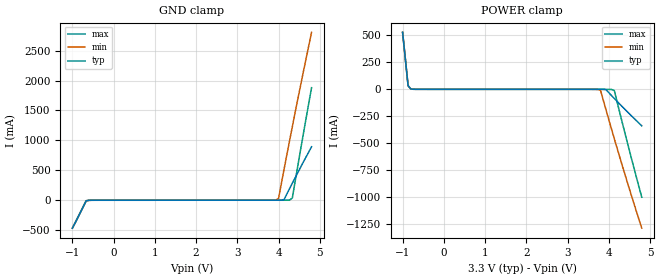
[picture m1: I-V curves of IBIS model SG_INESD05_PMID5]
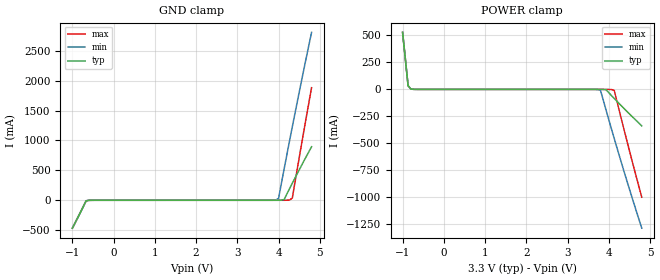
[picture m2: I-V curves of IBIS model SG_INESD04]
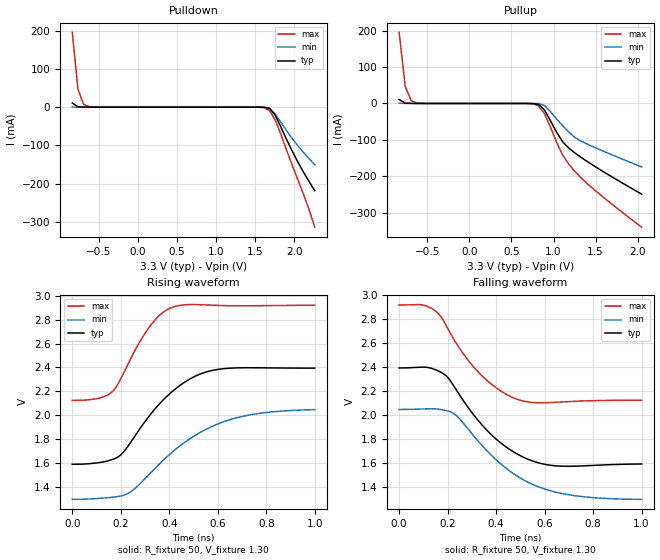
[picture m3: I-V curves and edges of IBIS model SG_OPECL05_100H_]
|   This file is an IBIS representation of the   |
|   Integrated Device Technology , Inc.   |
|   ICS853S310I   |
|   LOW SKEW 1-TO-8 DIFFERNTIAL-TO-3.3V LVPECL/ECL FANOUT BUFFER   |
[IBIS Ver]   4.1
[File name]   853s310i_3v3.ibs
[File Rev]   1.0
[Date]   29 Mar 2011
[Source]   Originated at Integrated Device Technology, Inc.
[Disclaimer]
IDT hereby grants the user of this IBIS model a non-exclusive,
nontransferable license to use this IBIS model under the following terms.
Before using this IBIS model, the user should read this license.
If the user does not accept these terms,  the IBIS model should be
returned to IDT within 30 days.
   The user is granted this license only to use the IBIS model and
is not granted rights to sell, load, rent, lease or license the IBIS
model in whole or in part, or in modified form to anyone other than
user. User may modify the IBIS model to suit its specific
applications but rights to derivative works and such modifications
shall belong to IDT.
   This IBIS model is provided on an "AS IS" basis and IDT makes
absolutely no warranty with respect to the information contained
herein. IDT DISCLAIMS AND CUSTOMER WAIVES ALL WARRANTIES, EXPRESS
OR IMPLIED, INCLUDING WARRANTIES OF MERCHANTABILITY OR FITNESS FOR
A PARTICULAR PURPOSE. The entire risk as to quality and performance
is with the Customer. ACCORDINGLY, IN NO EVENT SHALL THE COMPANY BE
LIABLE FOR ANY DAMAGES, WHETHER IN CONTRACT OR TORT,INCLUDING ANY
LOST PROFITS OR OTHER INCIDENTAL, CONSEQUENTIAL, EXEMPLARY, OR
PUNITIVE DAMAGES ARISING OUT OF THE USE OR APPLICATION OF THE IBIS
model provided in this package. Further, IDT reserves the right to
make changes without notice to any product herein to improve
reliability, function, or design. IDT does not convey any license
under patent rights or any other intellectual property rights,
including those of third parties.
   IDT is not obligated to provide maintenance or support
for the licensed IBIS model.
[Copyright]   Copyright 2011 by Integrated Device Technology , Inc.
[Component]   ICS53S310VI
[Manufacturer] Integrated Device Technology, Inc.
[Package]
|PLCC 28 Pin
|   typ   min   max
R_pkg   53.15m   49.2m   57.1m
L_pkg   3.123nH   2.878nH   3.368nH
C_pkg   0.65pF   0.632pF   0.667pF
[Pin] signal_name   model_name   R_pin   L_pin   C_pin
1   VCC   POWER   49.2m   2.878n   0.632p
2   nPCLK0   SG_INESD05_PMID5   51.2m   3.038n   0.643p
3   VBB   SG_INESD04   53.8m   3.201n   0.655p
4   PCLK1   SG_INESD05_PD75K   57.1m   3.368n   0.667p
5   nPCLK1   SG_INESD05_PMID5   57.1m   3.368n   0.667p
6   NC   NC   53.8m   3.201n   0.655p
7   nQ7   SG_OPECL05_100H_   51.2m   3.038n   0.643p
8   VCCO   POWER   49.2m   2.878n   0.632p
9   Q7   SG_OPECL05_100H_   51.2m   3.038n   0.643p
10   nQ6   SG_OPECL05_100H_   53.8m   3.201n   0.655p
11   Q6   SG_OPECL05_100H_   57.1m   3.368n   0.667p
12   nQ5   SG_OPECL05_100H_   57.1m   3.368n   0.667p
13   Q5   SG_OPECL05_100H_   53.8m   3.201n   0.655p
14   nQ4   SG_OPECL05_100H_   51.2m   3.038n   0.643p
15   VCCO   POWER   49.2m   2.878n   0.632p
16   Q4   SG_OPECL05_100H_   51.2m   3.038n   0.643p
17   nQ3   SG_OPECL05_100H_   53.8m   3.201n   0.655p
18   Q3   SG_OPECL05_100H_   57.1m   3.368n   0.667p
19   nQ2   SG_OPECL05_100H_   57.1m   3.368n   0.667p
20   Q2   SG_OPECL05_100H_   53.8m   3.201n   0.655p
21   nQ1   SG_OPECL05_100H_   51.2m   3.038n   0.643p
22   VCCO   POWER   49.2m   2.878n   0.632p
23   Q1   SG_OPECL05_100H_   51.2m   3.038n   0.643p
24   nQ0   SG_OPECL05_100H_   53.8m   3.201n   0.655p
25   Q0   SG_OPECL05_100H_   57.1m   3.368n   0.667p
26   VEE   GND   57.1m   3.368n   0.667p
27   CLK_SEL   SG_INESD05_PD75K   53.8m   3.201n   0.655p
28   PCLK0   SG_INESD05_PD75K   51.2m   3.038n   0.643p
[Diff Pin]  inv_pin  vdiff tdelay_typ tdelay_min  tdelay_max
|Input
28   2   0.15   0   0   0
4   5   0.15   0   0   0
|Output
9   7   NA   0   0   0
11   10   NA   0   0   0
13   12   NA   0   0   0
16   14   NA   0   0   0
18   17   NA   0   0   0
20   19   NA   0   0   0
23   21   NA   0   0   0
25   24   NA   0   0   0
| Models and submodels in the file (4): SG_INESD05_PMID5 (Input), SG_INESD04 (Input), SG_INESD05_PD75K (Input), SG_OPECL05_100H_ (Output_ECL)
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[Model]   SG_INESD05_PMID5
Model_type   Input
Polarity   Non-Inverting
Vinl = 0.8V
Vinh = 2.0V
|   typ   min   max
C_comp   2pF   1.5pF   2.5pF
|   typ   min   max
[Voltage range]   3.3V   3.135V   3.465V
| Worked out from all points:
|   GND clamp passes 1 mA (typ) near -0.57 V on its own axis
|   POWER clamp passes 1 mA (typ) near -0.75 V on its own axis
[GND_clamp]
|Voltage   I (typ)   I (min)   I (max)
-999mV    -466.2mA   -466.2mA   -466.2mA
-665.7mV  -9.075mA   -9.072mA   -9.078mA
-599.1mV  -1.392mA   -1.388mA   -1.395mA
3.867V    93.26uA    433uA      84.15uA
3.933V    121.1uA    2.991mA    87.1uA
4V        242.2uA    32.96mA    91.88uA
4.133V    10.39mA    518.4mA    165.1uA
4.267V    194mA      994.2mA    3.355mA
4.333V    284.5mA    1.229A     37.1mA
4.533V    550.4mA    1.918A     843mA
4.8V      892.8mA    2.805A     1.88A
[Power_clamp]
|Voltage   I (typ)   I (min)   I (max)
-999mV    527.8mA    527.8mA    527.8mA
-865.7mV  33.62mA    33.62mA    33.63mA
-799mV    3.051mA    3.048mA    3.054mA
3.6V      -77.29uA   -152.7uA   -73.6uA
3.8V      -251uA     -8.905mA   -82.96uA
3.933V    -3.316mA   -190.6mA   -165.6uA
4.133V    -84.48mA   -456.4mA   -9.953mA
4.467V    -214.4mA   -882mA     -517.4mA
4.8V      -338mA     -1.287A    -999.9mA
[Model]   SG_INESD04
Model_type   Input
Polarity   Non-Inverting
Vinl = 0.8V
Vinh = 2.0V
|   typ   min   max
C_comp   2pF   1.5pF   2.5pF
|   typ   min   max
[Voltage range]   3.3V   3.135V   3.465V
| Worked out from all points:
|   GND clamp passes 1 mA (typ) near -0.58 V on its own axis
|   POWER clamp passes 1 mA (typ) near -0.74 V on its own axis
[GND_clamp]
|Voltage   I (typ)   I (min)   I (max)
-999mV    -466.1mA   -466.1mA   -466.1mA
-665.7mV  -8.992mA   -8.992mA   -8.992mA
-599.1mV  -1.311mA   -1.311mA   -1.311mA
3.867V    60.84uA    520.1uA    51.14uA
3.933V    102.7uA    3.239mA    52.58uA
4V        278.2uA    33.38mA    57.05uA
4.133V    10.74mA    519.3mA    166.7uA
4.267V    194.7mA    995.5mA    3.61mA
4.333V    285.4mA    1.23A      37.53mA
4.533V    551.8mA    1.92A      844.1mA
4.8V      894.9mA    2.808A     1.882A
[Power_clamp]
|Voltage   I (typ)   I (min)   I (max)
-999mV    528.7mA    528.7mA    528.7mA
-865.7mV  34.05mA    34.05mA    34.05mA
-799mV    3.3mA      3.298mA    3.302mA
3.6V      -4.407uA   -78.79uA   -1.786uA
3.8V      -172.9uA   -8.826mA   -5.914uA
3.933V    -3.234mA   -190.5mA   -85.07uA
4.133V    -84.39mA   -456.3mA   -9.868mA
4.467V    -214.3mA   -881.9mA   -517.3mA
4.8V      -337.9mA   -1.287A    -999.8mA
[Model]   SG_OPECL05_100H_
Model_type   Output_ECL
Polarity   Non-Inverting
|   typ   min   max
C_comp   2pF   1.5pF   2.5pF
Vmeas = 1.99V
Rref = 50
Cref = 0
Vref = 1.3V
|   typ   min   max
[Voltage range]   3.3V   3.0V   3.8V
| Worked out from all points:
|   rising waveform, R_fixture 50, V_fixture 1.30: 20-80 % time 200ps typ, 277ps min, 132ps max; typ from 1.59 V to 2.4 V
|   falling waveform, R_fixture 50, V_fixture 1.30: 20-80 % time 200ps typ, 245ps min, 175ps max; typ from 2.39 V to 1.59 V
[Pulldown]
|Voltage   I (typ)   I (min)   I (max)
|Note, modeling breaks down at 250mA and above.  This is well beyond the functional   |
|operating range of the device.  Should this scenario occur, catastrophic failure and   |
|possible damage to the device and/or board is of higher concern than the I-V curve   |
|behavior.  The IBIS checker will flag currents in excess of 10A with warnings.  Lines   |
|with currents in excess of 0.35 A have been commented out.  The points still remain|
|available to the user if the user desires to use them.   |
|-3.04000e+00   1.92160e+08   2.51398e+08   1.39180e+08
|-2.78000e+00   1.62857e+08   2.13925e+08   1.17236e+08
|-2.52000e+00   1.33553e+08   1.76452e+08   9.52926e+07
|-2.26000e+00   1.04250e+08   1.38979e+08   7.33492e+07
|-2.00000e+00   7.49467e+07   1.01507e+08   5.14057e+07
|-1.99000e+00   7.38197e+07   1.00065e+08   5.05617e+07
|-1.91789e+00   6.56924e+07   8.96722e+07   4.44757e+07
|-1.84578e+00   5.75651e+07   7.92791e+07   3.83896e+07
|-1.77367e+00   4.94378e+07   6.88860e+07   3.23036e+07
|-1.70156e+00   4.13105e+07   5.84929e+07   2.62176e+07
|-1.62944e+00   3.31832e+07   4.80998e+07   2.01315e+07
|-1.55733e+00   2.50559e+07   3.77067e+07   1.40455e+07
|-1.48522e+00   1.69286e+07   2.73136e+07   7.95945e+06
|-1.41311e+00   8.80127e+06   1.69204e+07   2.03437e+06
|-1.34100e+00   1.34441e+06   6.52733e+06   2.48679e+05
|-1.26889e+00   8.12123e+04   2.80322e+05   3.04058e+04
|-1.19678e+00   4.91291e+03   7.75053e+03   3.72350e+03
|-1.12467e+00   3.01766e+02   2.18996e+02   4.60136e+02
|-1.05256e+00   2.05721e+01   7.44005e+00   5.93641e+01
|-9.80444e-01   1.45327e+00   2.48419e-01   8.49910e+00
|-9.08333e-01   1.25370e-01   8.96926e-03   1.15041e+00
-836.2mV  10.8mA     577.1uA    195.6mA
-764.1mV  1.014mA    102.6uA    46.98mA
-692mV    176.3uA    15.79uA    7.416mA
-619.9mV  34.19uA    1.702uA    1.157mA
1.543V    -16.52uA   -3.526uA   -181.8uA
1.616V    -258uA     -119.7uA   -1.382mA
1.688V    -3.483mA   -3.021mA   -8.864mA
1.76V     -21.46mA   -18.23mA   -33.6mA
1.832V    -52.26mA   -39.77mA   -71.71mA
2.048V    -143.4mA   -100.9mA   -189.5mA
2.192V    -194.7mA   -134.8mA   -268.5mA
2.265V    -218.1mA   -150.1mA   -313.8mA
| 2.33667e+00   -2.40431e-01   -1.64458e-01   -3.51948e-01
| 2.40878e+00   -2.60096e-01   -1.78057e-01   -3.86031e-01
| 2.48089e+00   -2.75926e-01   -1.90995e-01   -4.18389e-01
| 2.55300e+00   -2.90872e-01   -2.03400e-01   -4.50878e-01
| 2.62511e+00   -3.06643e-01   -2.14939e-01   -4.86417e-01
| 2.69722e+00   -3.23573e-01   -2.24622e-01   -5.12879e-01
| 2.76933e+00   -3.40823e-01   -2.33508e-01   -5.36910e-01
| 2.84144e+00   -3.57624e-01   -2.42318e-01   -5.60796e-01
| 2.91356e+00   -3.74840e-01   -2.51157e-01   -5.84860e-01
| 2.98567e+00   -3.92569e-01   -2.59837e-01   -6.08707e-01
| 3.05778e+00   -4.11772e-01   -2.68668e-01   -6.31533e-01
| 3.12989e+00   -4.26759e-01   -2.77928e-01   -6.53567e-01
| 3.20200e+00   -4.40899e-01   -2.86756e-01   -6.74897e-01
| 3.27411e+00   -4.55086e-01   -2.94483e-01   -6.95545e-01
| 3.34622e+00   -4.69164e-01   -3.01542e-01   -7.15540e-01
| 3.41833e+00   -4.82474e-01   -3.08477e-01   -7.34920e-01
| 3.49044e+00   -4.95288e-01   -3.15388e-01   -7.53730e-01
| 3.56256e+00   -5.07746e-01   -3.22427e-01   -7.72015e-01
| 3.63467e+00   -5.19904e-01   -3.29804e-01   -7.89818e-01
| 3.70678e+00   -5.31807e-01   -3.37709e-01   -8.07182e-01
| 3.77889e+00   -5.43539e-01   -3.52649e-01   -8.24146e-01
| 3.85100e+00   -5.55315e-01   -6.12529e-01   -8.40745e-01
| 3.92311e+00   -5.68261e-01   -8.64765e+00   -8.57014e-01
| 3.99522e+00   -5.99695e-01   -2.26919e+02   -8.72983e-01
| 4.06733e+00   -9.36993e-01   -8.00131e+03   -8.88690e-01
| 4.13944e+00   -6.03122e+00   -2.89295e+05   -9.04232e-01
| 4.21156e+00   -6.69016e+01   -1.76555e+06   -9.20172e-01
| 4.28367e+00   -1.03050e+03   -3.81856e+06   -9.40696e-01
| 4.35578e+00   -1.69373e+04   -1.33751e+07   -9.99273e-01
| 4.42789e+00   -2.80216e+05   -2.52525e+07   -1.36920e+00
| 4.50000e+00   -1.41833e+06   -3.71298e+07   -4.27555e+00
| 4.51000e+00   -1.58193e+06   -3.87769e+07   -5.29764e+00
| 4.92800e+00   -4.13220e+07   -1.07625e+08   -5.40432e+05
| 5.34600e+00   -9.51608e+07   -1.76474e+08   -1.86671e+07
| 5.76400e+00   -1.49000e+08   -2.45322e+08   -5.89836e+07
| 6.18200e+00   -2.02838e+08   -3.14171e+08   -9.93001e+07
| 6.60000e+00   -2.56677e+08   -3.83019e+08   -1.39617e+08
[Pullup]
|Voltage   I (typ)   I (min)   I (max)
|Note, modeling breaks down at 250mA and above.  This is well beyond the functional   |
|operating range of the device.  Should this scenario occur, catastrophic failure and   |
|possible damage to the device and/or board is of higher concern than the I-V curve   |
|behavior.  The IBIS checker will flag currents in excess of 10A with warnings.  Lines   |
|with currents in excess of 0.35 A have been commented out.  The points still remain|
|available to the user if the user desires to use them.   |
|-3.04000e+00   1.92160e+08   2.51398e+08   1.39180e+08
|-2.78000e+00   1.62857e+08   2.13925e+08   1.17236e+08
|-2.52000e+00   1.33553e+08   1.76452e+08   9.52926e+07
|-2.26000e+00   1.04250e+08   1.38979e+08   7.33492e+07
|-2.00000e+00   7.49467e+07   1.01507e+08   5.14057e+07
|-1.99000e+00   7.38197e+07   1.00065e+08   5.05617e+07
|-1.91789e+00   6.56924e+07   8.96722e+07   4.44757e+07
|-1.84578e+00   5.75651e+07   7.92791e+07   3.83896e+07
|-1.77367e+00   4.94378e+07   6.88860e+07   3.23036e+07
|-1.70156e+00   4.13105e+07   5.84929e+07   2.62176e+07
|-1.62944e+00   3.31832e+07   4.80998e+07   2.01315e+07
|-1.55733e+00   2.50559e+07   3.77067e+07   1.40455e+07
|-1.48522e+00   1.69286e+07   2.73136e+07   7.95945e+06
|-1.41311e+00   8.80127e+06   1.69204e+07   2.03437e+06
|-1.34100e+00   1.34441e+06   6.52733e+06   2.48679e+05
|-1.26889e+00   8.12123e+04   2.80322e+05   3.04058e+04
|-1.19678e+00   4.91291e+03   7.75053e+03   3.72350e+03
|-1.12467e+00   3.01766e+02   2.18996e+02   4.60136e+02
|-1.05256e+00   2.05721e+01   7.44005e+00   5.93641e+01
|-9.80444e-01   1.45327e+00   2.48419e-01   8.49910e+00
|-9.08333e-01   1.25370e-01   8.96926e-03   1.15041e+00
-836.2mV  10.8mA     577.1uA    195.6mA
-764.1mV  1.014mA    102.6uA    46.98mA
-692mV    176.3uA    15.79uA    7.416mA
-547.8mV  5.429uA    127.7nA    221.1uA
678.1mV   -11.66uA   -270.6nA   -129.6uA
822.3mV   -2.582mA   -309.3uA   -6.727mA
894.4mV   -18.47mA   -5.864mA   -28.68mA
1.039V    -79.75mA   -43.04mA   -107.5mA
1.111V    -105.9mA   -61.58mA   -142.6mA
1.255V    -136.3mA   -93.54mA   -187.1mA
1.543V    -180.5mA   -126.3mA   -248.5mA
2.048V    -249.3mA   -174.6mA   -340.2mA
| 2.12033e+00   -2.58738e-01   -1.81338e-01   -3.52687e-01
| 2.19244e+00   -2.68106e-01   -1.88047e-01   -3.65121e-01
| 2.26456e+00   -2.77414e-01   -1.94733e-01   -3.77501e-01
| 2.33667e+00   -2.86665e-01   -2.01400e-01   -3.90099e-01
| 2.40878e+00   -2.95864e-01   -2.08048e-01   -4.04251e-01
| 2.48089e+00   -3.05015e-01   -2.14679e-01   -4.22696e-01
| 2.55300e+00   -3.14121e-01   -2.21294e-01   -4.45830e-01
| 2.62511e+00   -3.23201e-01   -2.27895e-01   -4.72038e-01
| 2.69722e+00   -3.32382e-01   -2.34495e-01   -4.99750e-01
| 2.76933e+00   -3.42036e-01   -2.41162e-01   -5.27652e-01
| 2.84144e+00   -3.53278e-01   -2.47893e-01   -5.55138e-01
| 2.91356e+00   -3.67602e-01   -2.54635e-01   -5.81422e-01
| 2.98567e+00   -3.84318e-01   -2.61400e-01   -6.06033e-01
| 3.05778e+00   -4.01790e-01   -2.68528e-01   -6.29555e-01
| 3.12989e+00   -4.19446e-01   -2.76332e-01   -6.52157e-01
| 3.20200e+00   -4.36765e-01   -2.84447e-01   -6.73900e-01
| 3.27411e+00   -4.52262e-01   -2.92599e-01   -6.94839e-01
| 3.34622e+00   -4.66498e-01   -3.00258e-01   -7.15040e-01
| 3.41833e+00   -4.79967e-01   -3.07400e-01   -7.34563e-01
| 3.49044e+00   -4.92857e-01   -3.14433e-01   -7.53471e-01
| 3.56256e+00   -5.05273e-01   -3.21559e-01   -7.71822e-01
| 3.63467e+00   -5.17286e-01   -3.29002e-01   -7.89669e-01
| 3.70678e+00   -5.28958e-01   -3.36964e-01   -8.07058e-01
| 3.77889e+00   -5.40395e-01   -3.51967e-01   -8.24035e-01
| 3.85100e+00   -5.51837e-01   -6.11919e-01   -8.40638e-01
| 3.92311e+00   -5.64439e-01   -8.64712e+00   -8.56904e-01
| 3.99522e+00   -5.95567e-01   -2.26919e+02   -8.72864e-01
| 4.06733e+00   -9.32667e-01   -8.00131e+03   -8.88559e-01
| 4.13944e+00   -6.02690e+00   -2.89295e+05   -9.04085e-01
| 4.21156e+00   -6.68975e+01   -1.76555e+06   -9.20008e-01
| 4.28367e+00   -1.03049e+03   -3.81856e+06   -9.40514e-01
| 4.35578e+00   -1.69373e+04   -1.33751e+07   -9.99070e-01
| 4.42789e+00   -2.80216e+05   -2.52525e+07   -1.36897e+00
| 4.50000e+00   -1.41833e+06   -3.71298e+07   -4.27531e+00
| 4.51000e+00   -1.58193e+06   -3.87769e+07   -5.29739e+00
| 4.92800e+00   -4.13220e+07   -1.07625e+08   -5.40432e+05
| 5.34600e+00   -9.51608e+07   -1.76474e+08   -1.86671e+07
| 5.76400e+00   -1.49000e+08   -2.45322e+08   -5.89836e+07
| 6.18200e+00   -2.02838e+08   -3.14171e+08   -9.93001e+07
| 6.60000e+00   -2.56677e+08   -3.83019e+08   -1.39617e+08
[Ramp]
|   typ   min   max
dV/dt_r   0.483/0.201n   0.449/0.276n   0.48/0.133n
dV/dt_f   0.496/0.21n   0.453/0.245n   0.492/0.184n
R_load =   50.0000
[Rising Waveform]
R_fixture = 50
V_fixture = 1.30   | VCC_typ - 2V
V_fixture_max = 1.8   | VCC_max - 2V
V_fixture_min = 1.0   | VCC_min - 2V
C_fixture = 0.0p
| Time   typ   min   max
0s        1.592V     1.299V     2.125V
103.1ps   1.604V     1.306V     2.141V
163.2ps   1.63V      1.316V     2.195V
236.2ps   1.761V     1.356V     2.456V
312.3ps   1.982V     1.499V     2.722V
360.4ps   2.098V     1.598V     2.837V
409.4ps   2.194V     1.689V     2.9V
524.5ps   2.343V     1.855V     2.925V
652.7ps   2.395V     1.966V     2.915V
1ns       2.395V     2.048V     2.92V
[Falling Waveform]
R_fixture = 50
V_fixture = 1.30   | VCC_typ - 2V
V_fixture_max = 1.8   | VCC_max - 2V
V_fixture_min = 1.0   | VCC_min - 2V
C_fixture = 0.0p
| Time   typ   min   max
0s        2.394V     2.047V     2.92V
113.1ps   2.399V     2.053V     2.911V
157.2ps   2.373V     2.051V     2.858V
187.2ps   2.34V      2.041V     2.772V
238.2ps   2.202V     1.993V     2.591V
322.3ps   1.964V     1.791V     2.368V
477.5ps   1.686V     1.503V     2.14V
573.6ps   1.602V     1.402V     2.103V
676.7ps   1.573V     1.344V     2.111V
1ns       1.592V     1.297V     2.125V
